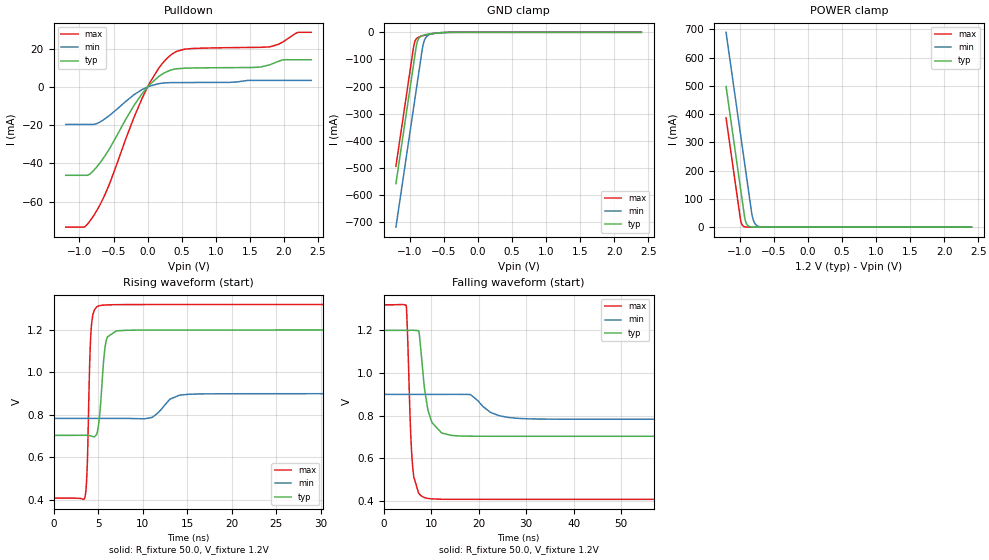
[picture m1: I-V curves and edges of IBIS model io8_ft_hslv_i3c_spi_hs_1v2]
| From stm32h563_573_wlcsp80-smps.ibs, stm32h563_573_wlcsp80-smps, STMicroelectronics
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[Model]   io8_ft_hslv_i3c_spi_hs_1v2
Model_type I/O_open_drain
Polarity   Non-Inverting
Enable   Active-Low
| CAP_THRESHOLD on pad IOFT is "UDTCAPC" :
| Rising=20.0% of vddiom   Falling=80.0% of vddiom
| C_comp min and max val. don't necessarily correlate with the min and max pvt
| but are the smallest and greatest pad capacitance found.
| var   typ   min   max
C_comp   3.41800pF  3.40005pF  3.42905pF
|C_comp_pulldown   3.41800pF  3.40005pF  3.42905pF
Vinl = 450.0mV
Vinh = 660.0mV
Vmeas = 600.0mV   | Reference voltage for timing measurements
Cref  = 50.0pF   | Timing specification test load capacitance value
Rref  = 1.0MOhm   | Timing specification test load resistance value
Vref  = 660.0mV   | Timing specification test load voltage
[Model Spec]
| TIME_THRESHOLD on pin ZII2CV11 is "CMOS" :
| Rising=40.0% of vdd   Falling=60.0% of vdd
Vinl 447.80000mV 344.80000mV 489.80000mV
Vinh 733.20000mV 535.20000mV 813.20000mV
| variable   typ   min   max
[Temperature Range] 25.0 125.0 -40.0
| variable   typ   min   max
[Voltage Range] 1.2V 900.0mV 1.32V
| variable   typ   min   max
[POWER Clamp Reference] 1.2V 900.0mV 1.32V
| variable   typ   min   max
[GND Clamp Reference] 0V 0V 0V
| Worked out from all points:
|   slope of the pulldown table from 0 to 0.18 V, typ, clamps not added: 30.6 ohm
|   GND clamp passes 1 mA (typ) near -0.52 V on its own axis
|   POWER clamp passes 1 mA (typ) near -0.84 V on its own axis
|   rising waveform, R_fixture 50.0, V_fixture 1.2V: 20-80 % time 549ps typ, 1.58ns min, 330ps max; typ from 0.704 V to 1.2 V
|   falling waveform, R_fixture 50.0, V_fixture 1.2V: 20-80 % time 1.79ns typ, 4.01ns min, 906ps max; typ from 1.2 V to 0.704 V
[POWER Clamp]
-1.2V     497.8mA    689.2mA    386.5mA
-990mV    140.8mA    332.2mA    29.53mA
-980mV    123.8mA    315.2mA    17.95mA
-960mV    89.81mA    281.2mA    6.634mA
-930mV    38.81mA    230.2mA    1.49mA
-900mV    12.07mA    179.2mA    334.8uA
-870mV    3.756mA    128.2mA    75.22uA
-820mV    536.4uA    44.98mA    6.246uA
-790mV    166.9uA    18.76mA    1.403uA
-750mV    35.18uA    5.846mA    191.8nA
-590mV    70.09nA    55uA       165.5pA
2.4V      0A         0A         0A
[GND Clamp]
-1.2V     -558.2mA   -719mA     -494.1mA
-940mV    -116.2mA   -277mA     -52.06mA
-930mV    -99.19mA   -260mA     -39.94mA
-900mV    -49.1mA    -209mA     -23.76mA
-880mV    -30.14mA   -175mA     -19.6mA
-850mV    -17.82mA   -124mA     -16.09mA
-810mV    -11.73mA   -56.78mA   -12.91mA
-780mV    -9.444mA   -28.21mA   -10.92mA
-740mV    -7.291mA   -13.16mA   -8.574mA
-640mV    -3.573mA   -4.171mA   -3.954mA
-380mV    -61.75uA   -230.3uA   -20.32uA
2.4V      3.863nA    718.4nA    150.6pA
| variable   typ   min   max
[Pullup Reference] 1.2V 900.0mV 1.32V
| variable   typ   min   max
[Pulldown Reference] 0V 0V 0V
[Pulldown]
-1.2V     -46.17mA   -19.62mA   -73.27mA
-930mV    -46.17mA   -19.62mA   -73.18mA
-770mV    -42.8mA    -19.41mA   -66.04mA
-570mV    -32.88mA   -15.18mA   -51.58mA
-80mV     -3.488mA   -1.363mA   -5.887mA
160mV     5.368mA    1.686mA    9.621mA
340mV     8.782mA    2.251mA    16.66mA
540mV     9.805mA    2.305mA    19.74mA
1.79V     11.53mA    3.428mA    20.94mA
1.98V     14.11mA    3.428mA    23.43mA
2.2V      14.2mA     3.428mA    28.44mA
2.4V      14.2mA     3.428mA    28.54mA
[Ramp]
dV/dt_r 297.78949mV/547.26652ps 69.89602mV/1.50852ns 547.12751mV/327.62413ps
dV/dt_f 297.80308mV/1.71625ns 69.92402mV/3.79354ns 547.13946mV/906.14325ps
R_load = 50.0
| Removed startup time: 0s 0s 0s  .
| Removed end time: 49.4ns.
[Rising Waveform]
R_fixture   = 50.0
V_fixture   = 1.2V
V_fixture_min = 900.0mV
V_fixture_max = 1.32V
0s        703.7mV    783.5mV    408.1mV
3.55ns    704mV      783.5mV    417.3mV
3.8ns     703.6mV    783.5mV    578.4mV
4.05ns    702.2mV    783.5mV    1.031V
4.2ns     700.7mV    783.5mV    1.19V
5ns       738.7mV    783.5mV    1.312V
5.85ns    1.137V     783.6mV    1.318V
7.05ns    1.196V     783.6mV    1.319V
15.15ns   1.2V       897mV      1.32V
49.4ns    1.2V       900mV      1.32V
| Removed startup time: 0s 0s 0s  .
| Removed end time: 99.4ns.
[Falling Waveform]
R_fixture   = 50.0
V_fixture   = 1.2V
V_fixture_min = 900.0mV
V_fixture_max = 1.32V
0s        1.2V       900mV      1.32V
4.75ns    1.2V       900mV      1.317V
5.65ns    1.201V     900mV      739.8mV
6.1ns     1.201V     900mV      562.5mV
7.4ns     1.196V     900mV      435.8mV
8.45ns    957.4mV    900mV      417.6mV
10.15ns   768.2mV    900mV      410.1mV
14.2ns    707.9mV    900.2mV    408.2mV
28.4ns    703.7mV    787.4mV    408.1mV
99.4ns    703.7mV    783.5mV    408.1mV
